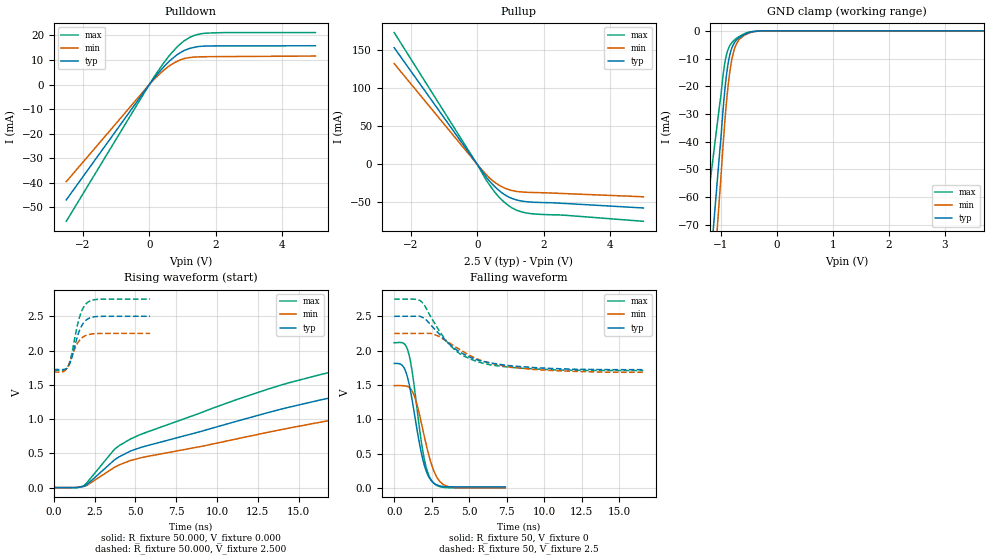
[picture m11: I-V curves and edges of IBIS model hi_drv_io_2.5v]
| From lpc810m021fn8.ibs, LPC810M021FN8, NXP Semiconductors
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[Model]   hi_drv_io_2.5v
Model_type I/O
Vinl=7.500E-01
Vinh=1.750E+00
Vref=0.000E+00
Rref=1.000E+06
Cref=2.000E-11
Vmeas=1.250E+00
C_comp   8.440E-13   8.280E-13   8.600E-13
[Voltage Range]   2.500E+00   2.250E+00   2.750E+00
[POWER Clamp Reference]   2.500E+00   2.250E+00   2.750E+00
[GND Clamp Reference]   0.000E+00   0.000E+00   0.000E+00
[Pullup Reference]   2.500E+00   2.250E+00   2.750E+00
[Pulldown Reference]   0.000E+00   0.000E+00   0.000E+00
[Temperature Range]   25   85   -40
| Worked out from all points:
|   slope of the pulldown table from 0 to 0.375 V, typ, clamps not added: 59.7 ohm
|   slope of the pullup table from 0 to 0.375 V, typ, clamps not added: 16.9 ohm
|   GND clamp passes 1 mA (typ) near -0.54 V on its own axis
|   rising waveform, R_fixture 50.000, V_fixture 0.000: 20-80 % time 16.4ns typ, 19.3ns min, 13.8ns max; typ from 0 V to 1.8 V
|   falling waveform, R_fixture 50, V_fixture 0: 20-80 % time 906ps typ, 1.01ns min, 800ps max; typ from 1.81 V to 0.017 V
|   rising waveform, R_fixture 50.000, V_fixture 2.500: 20-80 % time 594ps typ, 611ps min, 587ps max; typ from 1.72 V to 2.5 V
|   falling waveform, R_fixture 50, V_fixture 2.5: 20-80 % time 2.81ns typ, 3.33ns min, 2.37ns max; typ from 2.5 V to 1.72 V
[GND Clamp]
-2.5V     -404.4mA   -481mA     -268.3mA
-1.02V    -43.49mA   -58.74mA   -26.39mA
-1V       -39.04mA   -53.33mA   -23.63mA
-960mV    -28.39mA   -41.3mA    -16.04mA
-920mV    -19.57mA   -30.54mA   -10.58mA
-880mV    -13.05mA   -21.66mA   -7.23mA
-820mV    -7.167mA   -12.19mA   -4.716mA
-780mV    -5.099mA   -8.191mA   -3.748mA
-720mV    -3.33mA    -4.644mA   -2.706mA
-580mV    -1.348mA   -1.652mA   -1.054mA
-260mV    0A         0A         0A
5V        0A         0A         0A
[POWER Clamp]
-2.5V     0A         0A         0A
5V        0A         0A         0A
[Pullup]
-2.5V     153.2mA    132.3mA    173.1mA
0V        0A         0A         0A
180mV     -10.89mA   -9.091mA   -13.93mA
300mV     -18.43mA   -14.65mA   -22.66mA
540mV     -29.74mA   -23.99mA   -37.06mA
720mV     -36.56mA   -28.95mA   -45.88mA
920mV     -42.24mA   -32.74mA   -53.38mA
1.22V     -47.11mA   -35.71mA   -60.74mA
1.6V      -49.45mA   -36.84mA   -64.61mA
2.6V      -51.24mA   -38.3mA    -66.7mA
5V        -57.27mA   -42.56mA   -74.76mA
[Pulldown]
-2.5V     -46.95mA   -39.54mA   -55.67mA
140mV     2.506mA    2.066mA    3.025mA
420mV     6.967mA    5.639mA    8.535mA
620mV     9.719mA    7.744mA    12.05mA
840mV     12.14mA    9.477mA    15.36mA
1.04V     13.78mA    10.52mA    17.7mA
1.36V     15.14mA    11.18mA    19.99mA
1.7V      15.67mA    11.31mA    20.87mA
5V        15.74mA    11.58mA    21.14mA
[Rising Waveform]
R_fixture = 50.000
V_fixture = 0.000
V_fixture_min = 0.000
V_fixture_max = 0.000
|  time   V(typ)   V(min)   V(max)
0s        0V         0V         0V
1.8ns     15.77mV    15mV       23.48mV
3.7ns     400.6mV    293mV      554.5mV
5.4ns     590.4mV    437.7mV    782.4mV
13.8ns    1.136V     839.5mV    1.486V
19.1ns    1.408V     1.065V     1.783V
24.2ns    1.574V     1.223V     1.928V
31.1ns    1.687V     1.353V     2.017V
44.9ns    1.786V     1.464V     2.099V
53ns      1.798V     1.49V      2.111V
[Falling Waveform]
R_fixture = 50
V_fixture = 0
V_fixture_min = 0
V_fixture_max = 0
0s        1.814V     1.492V     2.114V
600ps     1.77V      1.489V     2.11V
1ns       1.507V     1.465V     1.932V
1.4ns     1.009V     1.303V     1.367V
1.9ns     421.3mV    856.4mV    544.2mV
2.2ns     209.7mV    568.8mV    248.2mV
2.5ns     100.2mV    333.8mV    104.8mV
3ns       33.43mV    106.3mV    23.2mV
3.6ns     18.27mV    22.11mV    4.521mV
7.4ns     17.15mV    4.571mV    2.64mV
[Rising Waveform]
R_fixture = 50.000
V_fixture = 2.500
V_fixture_min = 2.250
V_fixture_max = 2.750
|  time   V(typ)   V(min)   V(max)
0s        1.723V     1.685V     1.709V
600ps     1.723V     1.694V     1.713V
900ps     1.771V     1.783V     1.78V
1.1ns     1.895V     1.907V     1.952V
1.3ns     2.078V     2.034V     2.202V
1.6ns     2.309V     2.157V     2.508V
1.8ns     2.397V     2.2V       2.623V
2.1ns     2.463V     2.231V     2.708V
2.8ns     2.498V     2.249V     2.748V
5.9ns     2.5V       2.25V      2.75V
[Falling Waveform]
R_fixture = 50
V_fixture = 2.5
V_fixture_min = 2.25
V_fixture_max = 2.75
0s        2.5V       2.25V      2.75V
1.4ns     2.5V       2.25V      2.748V
1.8ns     2.493V     2.25V      2.715V
2.6ns     2.335V     2.244V     2.432V
3.8ns     2.071V     2.095V     2.06V
4.6ns     1.953V     1.985V     1.925V
5.8ns     1.849V     1.856V     1.824V
7.6ns     1.784V     1.765V     1.761V
9.3ns     1.754V     1.727V     1.735V
16.6ns    1.723V     1.685V     1.709V
[Ramp]
dV/dt_r   1.0783E+00/1.6358E-08   8.9218E-01/1.9294E-08   1.2670E+00/1.3882E-08
dV/dt_f   4.6607E-01/2.8065E-09   3.3898E-01/3.2420E-09   6.2439E-01/2.3520E-09
R_load = 50
